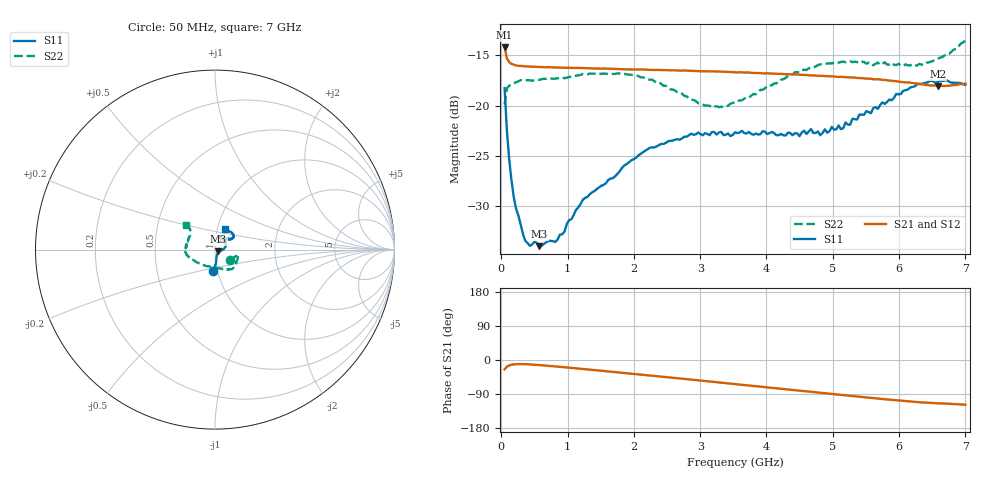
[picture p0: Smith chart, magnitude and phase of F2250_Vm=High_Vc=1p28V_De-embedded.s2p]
! Integrated Device Technology
! Corporate Headquarters
! 6024 Silver Creek Valley Road
! San Jose, CA 95138  USA
! Phone:  1-408-284-8200
! Toll Free:  1-800-223-1366
! Webpage:  http://www.idt.com/
! Timing and RF Division
! 515 Groton Road, Suite 102
! Westford, MA 01886-6024
! Device:  F2250
! Description: Voltage Variable RF Attenuator
! Frequency:  50.0 -  6000.00 MHz
! Package:  3x3 mm Thin QFN Plastic Package: 16 pin
! Ports:  2 RF, 3 DC
!  Pin  1  = GND
!  Pin  2  = NC
!  Pin  3  = RF1  = Port 1
!  Pin  4  = NC
!  Pin  5  = GND
!  Pin  6  = GND
!  Pin  7  = GND
!  Pin  8  = GND
!  Pin  9  = NC
!  Pin 10  = RF2  = Port 2
!  Pin 11  = NC
!  Pin 12  = GND
!  Pin 13  = GND
!  Pin 14  = VCNTRL
!  Pin 15  = VDD
!  Pin 16  = VMODE
! Vcntrl:  1.280 Volts
! Vmode:  +3.300 Volts
! Vdd:  +3.30  Volts
! Current:  1.331 mA
! Data:  The device was measured on a the F2250 evaluation board which has
!  individual transmission lines to the RF pins.  Data was collected
!  using a calibrated network analyzer.  The evaluation board was
!  de-embedded using a TRL calibration technique.
!  The reference plane is the edge of the package pin.
! Misc:  SN 10
!  Action Tracker AT0258
! Date Measured:  2014-11-26
! Date:  2015-10-15  MJV
! Note:
!  Integrated Device Technology supplies this data as a sample of measured
!  data at the package pin for this product.  Your particular data for this
!  product may vary.
!  Data was taken at 25 degrees C.
!  Integrated Device Technology reserves the right to change this data at anytime.
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# GHz S dB R 50
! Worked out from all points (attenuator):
!   201 points, 50 MHz to 7 GHz, reference 50 ohm
!   highest |S21| = -14.18 dB at 50 MHz (marker M1); lowest = -18.1 dB at 6.583 GHz (marker M2)
!   lowest |S11| = -34.0 dB at 571.2 MHz (marker M3), VSWR 1.04, Z = 51.8 - j0.942 ohm
!   |S11| at or under -10 dB: start of sweep to end of sweep
!   |S22| runs from -20.1 to -13.5 dB; largest |S21 - S12| = 0.00072
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0.05  -18.26 -95.2  -14.18 -24.5  -14.19 -24.5  -19.87 -36.1
0.08475  -22.52 -85.7  -15.29 -17.7  -15.29 -17.7  -18.29 -18.0
0.1195  -25.35 -82.1  -15.68 -14.3  -15.67 -14.3  -18.01 -13.2
0.189  -29.13 -72.6  -15.93 -11.5  -15.93 -11.5  -17.77 -11.8
0.22375  -30.25 -67.0  -16.00 -11.0  -16.00 -11.0  -17.67 -12.2
0.36275  -33.45 -48.4  -16.09 -11.1  -16.10 -11.1  -17.49 -13.4
0.57125  -33.97 -27.0  -16.16 -13.3  -16.16 -13.4  -17.44 -19.0
0.84925  -33.31 -18.5  -16.20 -17.5  -16.21 -17.5  -17.28 -27.1
1.2315  -29.33 -10.5  -16.26 -23.7  -16.26 -23.7  -16.85 -36.3
1.96125  -25.43 9.2  -16.40 -36.0  -16.39 -36.0  -16.93 -49.8
2.37825  -23.91 20.1  -16.45 -43.2  -16.44 -43.3  -17.64 -58.7
3.07325  -22.73 42.2  -16.57 -55.5  -16.56 -55.5  -19.99 -88.8
3.525  -22.65 56.8  -16.68 -63.5  -16.68 -63.5  -19.69 -119.3
4.7065  -22.72 65.3  -17.00 -84.6  -16.99 -84.6  -16.18 -166.5
5.15825  -22.24 47.9  -17.15 -92.6  -17.16 -92.6  -15.62 -176.0
5.193  -21.66 48.3  -17.17 -93.2  -17.17 -93.2  -15.67 -176.8
5.2625  -21.88 44.8  -17.19 -94.4  -17.18 -94.5  -15.58 -177.9
5.29725  -21.29 44.0  -17.20 -95.1  -17.19 -95.2  -15.67 -178.8
5.85325  -19.38 33.9  -17.51 -104.6  -17.50 -104.7  -15.91 167.2
6.27025  -17.89 34.6  -17.79 -111.1  -17.82 -111.1  -16.01 154.0
6.583  -17.63 41.4  -18.06 -114.3  -18.05 -114.4  -15.34 143.6
7  -17.92 62.8  -17.79 -118.0  -17.81 -118.1  -13.52 139.5
